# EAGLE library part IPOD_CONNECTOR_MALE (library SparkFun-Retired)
iPod Male Connector This is the connector that will insert into an iPods. Use this connector to gain access to the various iPod pins. Schematic and footprint are not yet production proven. The PCB thickness must be more thin than the standard 0.062" FR4. Spark Fun Electronics SKU : DEV-00633
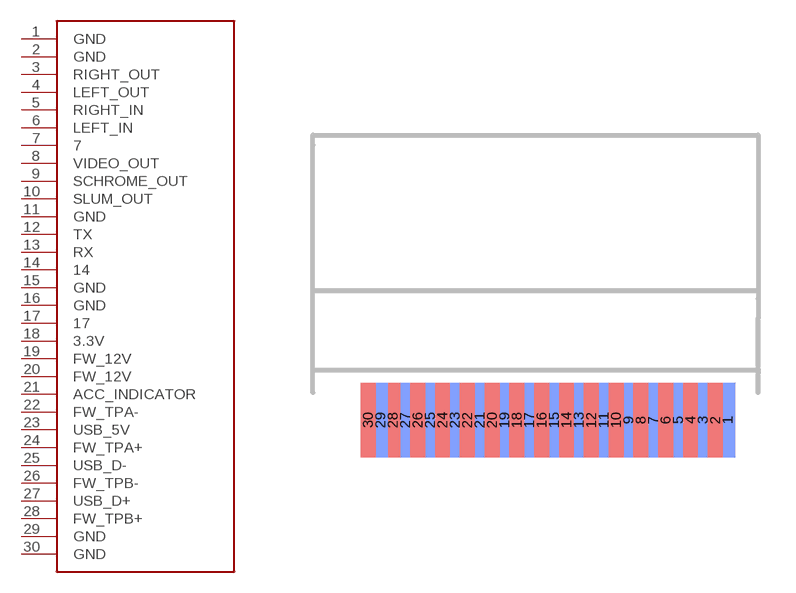
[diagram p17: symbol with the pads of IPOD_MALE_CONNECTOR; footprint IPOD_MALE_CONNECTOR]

Designator prefix -

## IPOD_CONNECTOR_MALE  [IPOD_MALE_CONNECTOR]
1  GND
2  GND
3  RIGHT_OUT
4  LEFT_OUT
5  RIGHT_IN
6  LEFT_IN
7  7
8  VIDEO_OUT
9  SCHROME_OUT
10  SLUM_OUT
11  GND
12  TX
13  RX
14  14
15  GND
16  GND
17  17
18  3.3V
19  FW_12V
20  FW_12V
21  ACC_INDICATOR
22  FW_TPA-
23  USB_5V
24  FW_TPA+
25  USB_D-
26  FW_TPB-
27  USB_D+
28  FW_TPB+
29  GND
30  GND

## Footprint IPOD_MALE_CONNECTOR (pad centres in mm)
smd 0.6 x 3 bottom: 1 7.5,0; 3 6.5,0; 5 5.5,0; 7 4.5,0; 9 3.5,0; 11 2.5,0; 13 1.5,0; 15 0.5,0; 17 -0.5,0; 19 -1.5,0; 21 -2.5,0; 23 -3.5,0; 25 -4.5,0; 27 -5.5,0; 29 -6.5,0
smd 0.6 x 3: 2 7,0; 4 6,0; 6 5,0; 8 4,0; 10 3,0; 12 2,0; 14 1,0; 16 0,0; 18 -1,0; 20 -2,0; 22 -3,0; 24 -4,0; 26 -5,0; 28 -6,0; 30 -7,0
